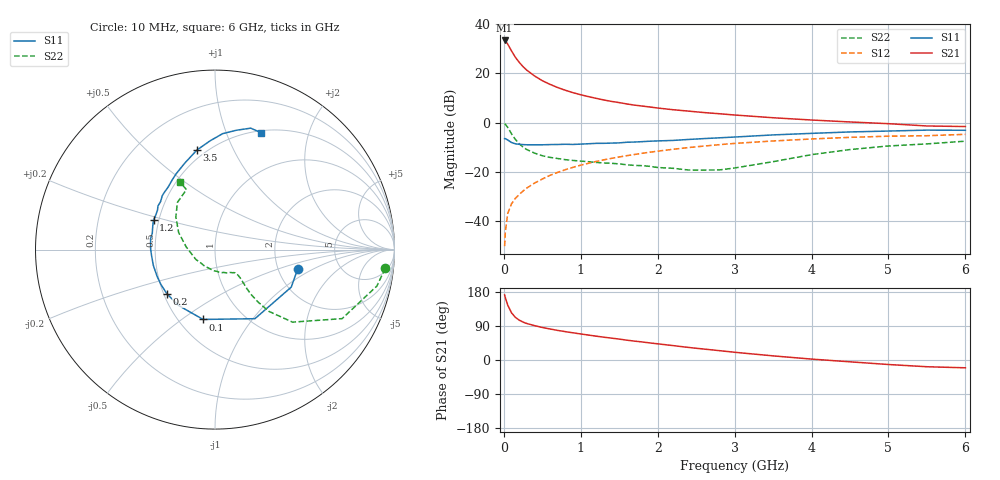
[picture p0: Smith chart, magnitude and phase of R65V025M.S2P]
! SIEMENS Small Signal Semiconductors
! BFR193
! Si NPN RF Bipolar Junction Transistor in SOT23
! VCE = 5 V  IC = 25 mA
! Common Emitter S-Parameters:  May  1996
# GHz  S  MA  R  50
!  f  S11  S21  S12  S22
! GHz  MAG  ANG  MAG  ANG  MAG  ANG  MAG  ANG
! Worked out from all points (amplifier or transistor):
!   36 points, 10 MHz to 6 GHz, reference 50 ohm
!   highest |S21| = 33.4 dB at 10 MHz (marker M1)
!   |S21| within 3 dB of that: start of sweep to 77.45 MHz
!   unconditionally stable (mu >= 1): 495.3 MHz to 1.883 GHz
!   at 250 MHz: K = 0.87, MSG = 25.3 dB, |S12| = -27.8 dB
!   at 1.4 GHz: K = 1.03, MAG = 10.6 dB, |S12| = -14.5 dB
!   at 6 GHz: K = 0.94, MSG = 1.6 dB, |S12| = -4.7 dB
!   S11 on the Smith chart (normalised r, x): 10 MHz: 2.55, -0.73; 100 MHz: 0.66, -0.60; 200 MHz: 0.52, -0.29; 1.2 GHz: 0.47, +0.18; 3.5 GHz: 0.45, +0.73; 6 GHz: 0.52, +1.34
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0.01  0.4729 -13.5  46.71 171.8  0.0031 86.6  0.9544 -6.3
0.02  0.4735 -26.2  45.49 164.2  0.0061 77.8  0.9243 -12.7
0.05  0.4446 -60.0  39.45 145.1  0.0142 71.0  0.8059 -28.5
0.1  0.3947 -99.7  28.61 124.5  0.0225 65.5  0.5915 -43.1
0.15  0.3716 -123.0  21.29 112.5  0.029 63.5  0.4564 -48.9
0.2  0.364 -137.5  16.8 105.2  0.0348 65.9  0.3738 -50.7
0.25  0.3583 -147.7  13.7 100.0  0.0409 66.7  0.318 -51.2
0.3  0.3554 -155.4  11.59 96.2  0.0471 68.1  0.2836 -50.8
0.4  0.3547 -166.0  8.862 90.7  0.0594 69.5  0.2403 -49.5
0.5  0.3551 -174.8  7.122 85.8  0.0716 70.3  0.2128 -48.4
0.6  0.3586 179.6  5.993 81.9  0.085 70.2  0.1971 -48.0
0.7  0.3604 174.5  5.171 78.1  0.0979 70.1  0.1868 -48.2
0.8  0.3639 170.3  4.541 74.8  0.1109 69.3  0.1771 -48.8
1.1  0.3729 158.2  3.379 65.8  0.1497 66.7  0.161 -53.2
1.2  0.38 154.1  3.116 62.9  0.1629 65.8  0.1557 -55.1
1.6  0.4002 142.5  2.395 52.3  0.2137 60.8  0.1394 -66.8
2.2  0.4356 126.7  1.831 38.0  0.2879 52.6  0.1182 -93.7
2.8  0.4921 112.9  1.518 24.7  0.357 43.7  0.1095 -138.9
3.5  0.5637 100.3  1.258 10.9  0.4245 32.9  0.1613 174.6
4.5  0.6475 86.2  1.033 -4.8  0.5033 18.7  0.2843 140.1
5.5  0.7053 73.6  0.856 -17.8  0.5429 4.6  0.3702 115.5
6  0.6999 68.4  0.834 -20.6  0.5793 0.6  0.4206 117.2
